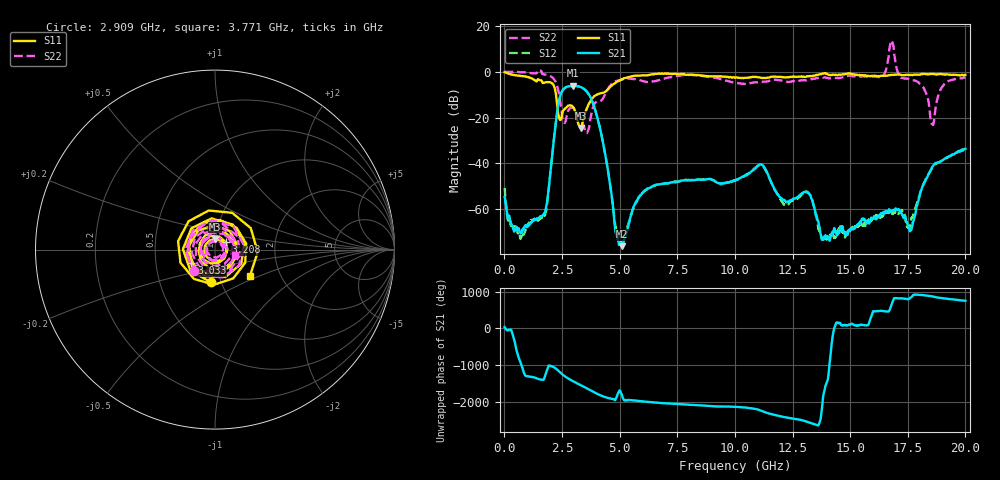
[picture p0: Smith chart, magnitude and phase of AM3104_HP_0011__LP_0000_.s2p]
!Created with skrf (http://scikit-rf.org).
# Hz S RI R 50.0
!freq ReS11 ImS11 ReS21 ImS21 ReS12 ImS12 ReS22 ImS22
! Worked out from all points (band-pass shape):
!   1601 points, 10 MHz to 20 GHz, reference 50 ohm
!   highest |S21| = -6.15 dB at 2.984 GHz (marker M1); lowest = -76.2 dB at 5.107 GHz (marker M2)
!   |S21| within 3 dB of the highest: 2.473 GHz to 3.614 GHz (1.141 GHz wide, 37.5 % of centre)
!   lowest |S11| = -24.5 dB at 3.321 GHz (marker M3), VSWR 1.13, Z = 49.6 + j5.91 ohm
!   |S11| at or under -10 dB: 2.239 GHz to 4.023 GHz (1.784 GHz wide, 57 % of centre)
!   |S22| runs from -26.8 to 13.6 dB; largest |S21 - S12| = 0.027
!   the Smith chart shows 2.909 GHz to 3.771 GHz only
!   S11 on the Smith chart (normalised r, x): 2.909 GHz: 0.89, -0.33; 3.033 GHz: 0.76, -0.12; 3.208 GHz: 1.12, +0.09; 3.771 GHz: 1.40, -0.44
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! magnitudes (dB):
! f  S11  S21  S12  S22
! 10 MHz  -0.2  -54.7  -50.7  0.0
! 672.2 MHz  -1.8  -70.1  -72.0  -0.2
! 1.709 GHz  -4.8  -62.1  -62.7  -1.1
! 2.384 GHz  -20.3  -12.1  -12.2  -10.6
! 2.909 GHz  -14.8  -6.3  -6.3  -15.6
! 2.984 GHz  -15.5  -6.1  -6.2  -15.9
! 3.033 GHz  -16.4  -6.2  -6.2  -16.1
! 3.208 GHz  -22.8  -6.4  -6.5  -18.6
! 3.321 GHz  -24.5  -6.8  -6.9  -20.0
! 3.346 GHz  -24.3  -6.9  -7.0  -20.7
! 3.771 GHz  -12.3  -11.9  -12.0  -18.7
! 5.107 GHz  -3.3  -76.2  -74.9  -3.4
! 6.682 GHz  -0.9  -49.2  -49.2  -3.8
! 10.01 GHz  -2.6  -47.6  -47.6  -4.8
! 11.14 GHz  -2.7  -40.6  -40.7  -4.5
! 12.15 GHz  -2.5  -56.1  -58.0  -4.1
! 13.34 GHz  -2.0  -55.7  -55.9  -3.3
! 13.85 GHz  -0.8  -73.2  -72.1  -2.5
! 16.68 GHz  -1.5  -60.1  -61.7  7.2
! 17.63 GHz  -1.4  -69.0  -65.6  -3.5
! 18.56 GHz  -0.9  -41.5  -41.9  -23.0
! 20 GHz  -1.4  -33.7  -33.4  -2.5
